[IBIS Ver]   4.1
[File Name]   sprm793.ibs
[File Rev]   1.0
[Date]   October 18, 2021
[Source]   File originated at Texas Instruments
[Copyright]   (c) 2012, Texas Instruments Inc.
[Component]   f771860xpn
[Manufacturer] Texas Instruments
[Package]
| Variable   Typ   Min   Max
R_pkg   0.197   0.066   0.282
L_pkg   5.76E-09   4.83E-09   7.44E-09
C_pkg   5.65E-13   4.94E-13   6.62E-13
[Pin]   signal_name   model_name   R_pin   L_Pin   C_Pin
1   GPIO30   BCF3385DSHYPBFZ_USF   2.28E-01   6.53746E-09   5.01E-13
2   GPIO31   BCF3385DSHYPBFZ_USF   2.23E-01   6.29611E-09   6.20E-13
3   GPIO29   BCPF335585DSHYPBFZ   2.07E-01   5.98591E-09   5.90E-13
4   GPIO28   BCF3385DSHYPBFZ_USF   2.03E-01   5.80933E-09   5.73E-13
5   XRSN   BQ0491FS_USF   1.97E-01   5.5995E-09   5.64E-13
6   GPIO46   BCF3385DSHYPBFZ_USF   1.93E-01   5.44478E-09   5.42E-13
7   VDDIO   NC   1.97E-01   5.44174E-09   5.21E-13
8   VDD   NC   1.98E-01   5.37212E-09   5.13E-13
9   VSS   NC   1.99E-01   5.35446E-09   4.94E-13
10   A6   ICF33SHYPB_USF   2.08E-01   5.46586E-09   5.09E-13
11   B2/C6   ICF33SHYPB_USF   2.02E-01   5.33465E-09   5.36E-13
12   A3/B3/VDAC,C5   ICF33SHYPB_USF   2.13E-01   5.3973E-09   5.94E-13
13   A2/B6/C9   ICF33SHYPB_USF   1.95E-01   5.30133E-09   5.33E-13
14   A15/B9/C7   ICF33SHYPB_USF   1.93E-01   5.35715E-09   5.62E-13
15   A14/B14/C4   ICF33SHYPB_USF   1.91E-01   5.40631E-09   5.42E-13
16   A11/B10/C0   ICF33SHYPB_USF   1.92E-01   5.5337E-09   5.60E-13
17   A5/B12/C2   ICF33SHYPB_USF   1.97E-01   5.71973E-09   6.13E-13
18   A1/B7/DACB_OUT   ICF33SHYPB_USF   2.02E-01   5.88825E-09   6.01E-13
19   A0/B15/C15/DACA_OUT   ICF33SHYPB_USF   2.11E-01   6.15795E-09   6.17E-13
20   VREFHI   NC   7.47E-02   5.62314E-09   5.45E-13
21   VREFLO   NC   7.39E-02   5.63782E-09   5.36E-13
22   A12,C1   ICF33SHYPB_USF   2.06E-01   6.09962E-09   6.35E-13
23   A7/C3   ICF33SHYPB_USF   2.02E-01   5.90043E-09   5.81E-13
24   A8/B0/C11   ICF33SHYPB_USF   1.93E-01   5.68909E-09   6.08E-13
25   VSSA   NC   6.89E-02   4.94081E-09   6.33E-13
26   VDDA   NC   6.61E-02   4.82658E-09   5.93E-13
27   A4/B8/C14   ICF33SHYPB_USF   1.88E-01   5.35512E-09   5.45E-13
28   A9/B4/C8   ICF33SHYPB_USF   1.92E-01   5.2817E-09   5.53E-13
29   A10/B1/C10   ICF33SHYPB_USF   1.89E-01   5.20421E-09   4.99E-13
30   VSS   NC   1.03E-01   4.92899E-09   5.35E-13
31   VDD   NC   1.01E-01   4.85871E-09   5.58E-13
32   VDDIO   NC   2.10E-01   5.35964E-09   5.76E-13
33   B5/GPIO20   BCF3385DSHYPBFZ   1.92E-01   5.27237E-09   5.26E-13
34   B11/GPIO21   BCF3385DSHYPBFZ   1.90E-01   5.32308E-09   5.16E-13
35   GPIO13   BCF3385DSHYPBFZ_USF   1.86E-01   5.27638E-09   5.13E-13
36   GPIO12   BCF3385DSHYPBFZ_USF   1.84E-01   5.32902E-09   5.41E-13
37   GPIO11   BCF3385DSHYPBFZ_USF   1.82E-01   5.40906E-09   5.60E-13
38   GPIO33   BCPF335585DSHYPBFZ   1.95E-01   5.73987E-09   5.85E-13
39   GPIO16   BCF3385DSHYPBFZ   2.16E-01   6.20938E-09   6.12E-13
40   GPIO17   BCF3385DSHYPBFZ   2.33E-01   6.55724E-09   5.04E-13
41   GPIO24   BCPF335585DSHYPBFZ   2.39E-01   6.71314E-09   5.09E-13
42   GPIO25   BCF3385DSHYPBFZ   2.26E-01   6.41211E-09   6.20E-13
43   GPIO26   BCF3385DSHYPBFZ   2.17E-01   6.14751E-09   5.89E-13
44   GPIO27   BCF3385DSHYPBFZ   2.14E-01   5.99079E-09   5.72E-13
45   TCK   BCF3355DSHYPBFZ_TMS_USF   2.07E-01   5.78366E-09   5.60E-13
46   GPIO37/TDO   BCPF335585DSHYPBFZ   2.02E-01   5.61292E-09   5.37E-13
47   TMS   BCF3355DSHYPBFZ_TMS_USF   2.00E-01   5.50275E-09   5.20E-13
48   GPIO35/TDI   BCF3385DSHYPBFZ   1.99E-01   5.38976E-09   5.21E-13
49   GPIO32   BCPF335585DSHYPBFZ   1.99E-01   5.35876E-09   5.01E-13
50   GPIO18/X2   BCPF335585DSHYPBFZ   2.03E-01   5.39832E-09   5.37E-13
51   GPIO19/X1   BCF3385DSHYPBFZ   2.15E-01   5.41779E-09   5.76E-13
52   VDDIO   NC   1.90E-01   5.31964E-09   6.08E-13
53   VDD   NC   9.70E-02   4.90095E-09   6.11E-13
54   GPIO43   BCF3385DSHYPBFZ_USF   1.92E-01   5.33634E-09   5.39E-13
55   VSS   NC   9.85E-02   5.0211E-09   6.37E-13
56   GPIO39   BCF3385DSHYPBFZ_USF   1.90E-01   5.48324E-09   5.54E-13
57   GPIO42   BCF3385DSHYPBFZ_USF   1.92E-01   5.60814E-09   5.57E-13
58   GPIO8   BCF3385DSHYPBFZ_USF   2.08E-01   5.98412E-09   5.91E-13
59   GPIO4   BCF3385DSHYPBFZ_USF   2.30E-01   6.45592E-09   6.22E-13
60   GPIO3   BCF3385DSHYPBFZ_USF   2.55E-01   6.94339E-09   5.19E-13
61   GPIO2   BCF3385DSHYPBFZ   2.82E-01   7.44202E-09   5.40E-13
62   GPIO1   BCPF335585DSHYPBFZ   2.67E-01   7.09004E-09   6.62E-13
63   GPIO0   BCF3385DSHYPBFZ   2.55E-01   6.77973E-09   6.22E-13
64   GPIO40   BCF3385DSHYPBFZ_USF   2.51E-01   6.60866E-09   6.03E-13
65   GPIO23   BCF3385DSHYPBFZ_USF   2.41E-01   6.3491E-09   5.94E-13
66   GPIO41   BCF3385DSHYPBFZ_USF   2.34E-01   6.14633E-09   5.65E-13
67   GPIO22   BCF3385DSHYPBFZ_USF   2.30E-01   5.99979E-09   5.46E-13
68   GPIO7   BCF3385DSHYPBFZ_USF   2.27E-01   5.85637E-09   5.46E-13
69   GPIO44   BCF3385DSHYPBFZ_USF   2.25E-01   5.7901E-09   5.39E-13
70   VSS   NC   1.26E-01   5.36393E-09   6.19E-13
71   VDD   NC   1.27E-01   5.24791E-09   6.51E-13
72   VDDIO   NC   2.29E-01   5.82525E-09   5.91E-13
73   GPIO45   BCF3385DSHYPBFZ_USF   2.22E-01   5.77087E-09   5.50E-13
74   GPIO5   BCF3385DSHYPBFZ_USF   2.21E-01   5.83186E-09   5.48E-13
75   GPIO9   BCF3385DSHYPBFZ_USF   2.21E-01   5.91152E-09   5.47E-13
76   GPIO10   BCF3385DSHYPBFZ_USF   2.20E-01   5.9869E-09   5.67E-13
77   GPIO34   BCF3385DSHYPBFZ_USF   2.23E-01   6.14485E-09   5.92E-13
78   GPIO15   BCF3385DSHYPBFZ_USF   2.29E-01   6.34468E-09   6.07E-13
79   GPIO14   BCF3385DSHYPBFZ_USF   2.33E-01   6.52601E-09   6.15E-13
80   GPIO6   BCF3385DSHYPBFZ_USF   2.37E-01   6.63529E-09   5.02E-13
| End of package information
|   Component IQ0440FS_VREGENZ_USF
[Component]   IQ0440FS_VREGENZ_USF
[Manufacturer]   Texas Instruments
[Package]
|  variable   typ   min   max
R_pkg   0   0   0
L_pkg   0   0   0
C_pkg   0   0   0
[Pin]   signal_name   model_name   R_pin   L_pin   C_pin
VSS   VSS   GND
VDDS   VDDS   POWER
PAD   PAD   IQ0440FS_VREGENZ_USF
[Model Selector] IQ0440FS_VREGENZ_USF
VREGENZ_WK_PD_ON_3P3  Cell operated at 3.3(nom)
|VREGENZ_WK_PD_ON_3P3; WEAK_PULLDOWN_ON
VREGENZ_WK_PD_OFF_3P3  Cell operated at 3.3(nom)
|   Component ICF33SHYPB_USF
[Component]   ICF33SHYPB_USF
[Manufacturer]   Texas Instruments
[Package]
|  variable   typ   min   max
R_pkg   0   0   0
L_pkg   0   0   0
C_pkg   0   0   0
[Pin]   signal_name   model_name   R_pin   L_pin   C_pin
VSS   VSS   GND
VDDS   VDDS   POWER
PAD   PAD   ICF33SHYPB_USF
[Model Selector] ICF33SHYPB_USF
ICF_WK_PUPD_OFF_3P3  Cell operated at 3.3(nom)
|ICF_WK_PUPD_OFF_3P3; WEAK_PULL_OFF
ICF_WK_PU_ON_3P3  Cell operated at 3.3(nom)
|ICF_WK_PU_ON_3P3; WEAK_PULLUP_ON
ICF_WK_PD_ON_3P3  Cell operated at 3.3(nom)
|   Component ICF33SHYPB_FS_SFII_CUS
[Component]   ICF33SHYPB_FS_SFII_CUS
[Manufacturer]   Texas Instruments
[Package]
|  variable   typ   min   max
R_pkg   0   0   0
L_pkg   0   0   0
C_pkg   0   0   0
[Pin]   signal_name   model_name   R_pin   L_pin   C_pin
VSS   VSS   GND
VDDS   VDDS   POWER
PAD   PAD   ICF33SHYPB_FS_SFII_CUS
[Model Selector] ICF33SHYPB_FS_SFII_CUS
CUS_WK_PUPD_OFF_3P3  Cell operated at 3.3(nom)
|CUS_WK_PUPD_OFF_3P3; WEAK_PULL_OFF
CUS_WK_PU_ON_3P3  Cell operated at 3.3(nom)
|CUS_WK_PU_ON_3P3; WEAK_PULLUP_ON
CUS_WK_PD_ON_3P3  Cell operated at 3.3(nom)
|   Component BT3308BT5FSHYPB_SFII
[Component]   BT3308BT5FSHYPB_SFII
[Manufacturer]   Texas Instruments
[Package]
|  variable   typ   min   max
R_pkg   0   0   0
L_pkg   0   0   0
C_pkg   0   0   0
[Pin]   signal_name   model_name   R_pin   L_pin   C_pin
VSS   VSS   GND
VDDS   VDDS   POWER
PAD   PAD   BT3308BT5FSHYPB_SFII
[Model Selector] BT3308BT5FSHYPB_SFII
BT_OPEN_DRAIN_6MA_3P3  Cell operated at 3.3(nom)
|BT_OPEN_DRAIN_6MA_3P3
BT_WEAK_PD_ON_3P3  Cell operated at 3.3(nom)
|BT_WEAK_PD_ON_3P3
BT_OPEN_DRAIN_3MA_3P3  Cell operated at 3.3(nom)
|BT_OPEN_DRAIN_3MA_3P3
BT_DRIVER_MODE_6MA_3P3  Cell operated at 3.3(nom)
|BT_DRIVER_MODE_6MA_3P3
BT_DRIVER_MODE_3MA_3P3  Cell operated at 3.3(nom)
|BT_DRIVER_MODE_3MA_3P3
BT_WEAK_PU_ON_3P3  Cell operated at 3.3(nom)
|   Component BQ0491FS_USF
[Component]   BQ0491FS_USF
[Manufacturer]   Texas Instruments
[Package]
|  variable   typ   min   max
R_pkg   0   0   0
L_pkg   0   0   0
C_pkg   0   0   0
[Pin]   signal_name   model_name   R_pin   L_pin   C_pin
VSS   VSS   GND
VDDS   VDDS   POWER
PAD   PAD   BQ0491FS_USF
[Model Selector] BQ0491FS_USF
XRSN_WK_PU_ON_3P3  Cell operated at 3.3(nom)
|XRSN_WK_PU_ON_3P3; WEAK_PULLUP_ON
XRSN_OPEN_DRAIN  Cell operated at 3.3(nom)
|   Component BCPF335585DSHYPBFZ
[Component]   BCPF335585DSHYPBFZ
[Manufacturer]   Texas Instruments
[Package]
|  variable   typ   min   max
R_pkg   0   0   0
L_pkg   0   0   0
C_pkg   0   0   0
[Pin]   signal_name   model_name   R_pin   L_pin   C_pin
VSS   VSS   GND
VDDS   VDDS   POWER
PAD   PAD   BCPF335585DSHYPBFZ
[Model Selector] BCPF335585DSHYPBFZ
BCPF_WK_PU_ON_3P3  Cell operated at 3.3(nom)
|BCPF_WK_PU_ON_3P3; WEAK_PULLUP_ON
BCPF_DRIVER_4MA_3P3  Cell operated at 3.3(nom)
|BCPF_DRIVER_4MA_3P3
BCPF_DRIVER_2MA_3P3  Cell operated at 3.3(nom)
|BCPF_DRIVER_2MA_3P3
BCPF_WK_PD_ON_3P3  Cell operated at 3.3(nom)
|   Component BCF3385DSHYPBFZ_USF
[Component]   BCF3385DSHYPBFZ_USF
[Manufacturer]   Texas Instruments
[Package]
|  variable   typ   min   max
R_pkg   0   0   0
L_pkg   0   0   0
C_pkg   0   0   0
[Pin]   signal_name   model_name   R_pin   L_pin   C_pin
VSS   VSS   GND
VDDS   VDDS   POWER
PAD   PAD   BCF3385DSHYPBFZ_USF
[Model Selector] BCF3385DSHYPBFZ_USF
BCF3385DUSF_WK_PU  Cell operated at 3.3(nom)
| BCF3385DUSF_WK_PU; WEAK_PULLUP_ON
BCF3385DUSF_DRIVER_3P3  Cell operated at 3.3(nom)
|BCF3385DUSF_DRIVER_3P3
BCF3385DUSF_WK_PD  Cell operated at 3.3(nom)
|   Component BCF3385DSHYPBFZ
[Component]   BCF3385DSHYPBFZ
[Manufacturer]   Texas Instruments
[Package]
|  variable   typ   min   max
R_pkg   0   0   0
L_pkg   0   0   0
C_pkg   0   0   0
[Pin]   signal_name   model_name   R_pin   L_pin   C_pin
VSS   VSS   GND
VDDS   VDDS   POWER
PAD   PAD   BCF3385DSHYPBFZ
[Model Selector] BCF3385DSHYPBFZ
BCF3385D_WK_PU_3P3  Cell operated at 3.3(nom)
|BCF3385D_WK_PU_3P3; WEAK_PULLUP_ON
BCF3385D_DRIVER_3P3  Cell operated at 3.3(nom)
|BCF3385D_DRIVER_3P3
BCF3385D_WK_PD_3P3  Cell operated at 3.3(nom)
|   Component BCF3355DSHYPBFZ_TMS_USF
[Component]   BCF3355DSHYPBFZ_TMS_USF
[Manufacturer]   Texas Instruments
[Package]
|  variable   typ   min   max
R_pkg   0   0   0
L_pkg   0   0   0
C_pkg   0   0   0
[Pin]   signal_name   model_name   R_pin   L_pin   C_pin
VSS   VSS   GND
VDDS   VDDS   POWER
PAD   PAD   BCF3355DSHYPBFZ_TMS_USF
[Model Selector] BCF3355DSHYPBFZ_TMS_USF
TMS_WK_PU_ON_3P3  Cell operated at 3.3(nom)
|TMS_WK_PU_ON_3P3; WEAK_PULLUP_ON
TMS_DRIVER_3P3  Cell operated at 3.3(nom)
|TMS_DRIVER_3P3
TMS_WK_PD_ON_3P3  Cell operated at 3.3(nom)
|   Component BCF3335DSHYPBFZ
[Component]   BCF3335DSHYPBFZ
[Manufacturer]   Texas Instruments
[Package]
|  variable   typ   min   max
R_pkg   0   0   0
L_pkg   0   0   0
C_pkg   0   0   0
[Pin]   signal_name   model_name   R_pin   L_pin   C_pin
VSS   VSS   GND
VDDS   VDDS   POWER
PAD   PAD   BCF3335DSHYPBFZ
[Model Selector] BCF3335DSHYPBFZ
BCF3335D_WK_PU_3P3  Cell operated at 3.3(nom)
|BCF3335D_WK_PU_3P3; WEAK_PULLUP_ON
BCF3335D_DRIVER_3P3  Cell operated at 3.3(nom)
|BCF3335D_DRIVER_3P3
BCF3335D_WK_PD_3P3  Cell operated at 3.3(nom)
| Models and submodels in the file (32): VREGENZ_WK_PD_ON_3P3 (Input), VREGENZ_WK_PD_OFF_3P3 (Input), ICF_WK_PUPD_OFF_3P3 (Input), ICF_WK_PU_ON_3P3 (Input), ICF_WK_PD_ON_3P3 (Input), CUS_WK_PUPD_OFF_3P3 (Input), CUS_WK_PU_ON_3P3 (Input), CUS_WK_PD_ON_3P3 (Input), BT_OPEN_DRAIN_6MA_3P3 (I/O_open_drain), BT_WEAK_PD_ON_3P3 (Input), BT_OPEN_DRAIN_3MA_3P3 (I/O_open_drain), BT_DRIVER_MODE_6MA_3P3 (I/O), BT_DRIVER_MODE_3MA_3P3 (I/O), BT_WEAK_PU_ON_3P3 (Input), XRSN_WK_PU_ON_3P3 (Input), XRSN_OPEN_DRAIN (I/O_open_drain), BCPF_WK_PU_ON_3P3 (Input), BCPF_DRIVER_4MA_3P3 (I/O), BCPF_DRIVER_2MA_3P3 (I/O), BCPF_WK_PD_ON_3P3 (Input), BCF3385DUSF_WK_PU (Input), BCF3385DUSF_DRIVER_3P3 (I/O), BCF3385DUSF_WK_PD (Input), BCF3385D_WK_PU_3P3 (Input), BCF3385D_DRIVER_3P3 (I/O), BCF3385D_WK_PD_3P3 (Input), TMS_WK_PU_ON_3P3 (Input), TMS_DRIVER_3P3 (I/O), TMS_WK_PD_ON_3P3 (Input), BCF3335D_WK_PU_3P3 (Input), BCF3335D_DRIVER_3P3 (I/O), BCF3335D_WK_PD_3P3 (Input)
